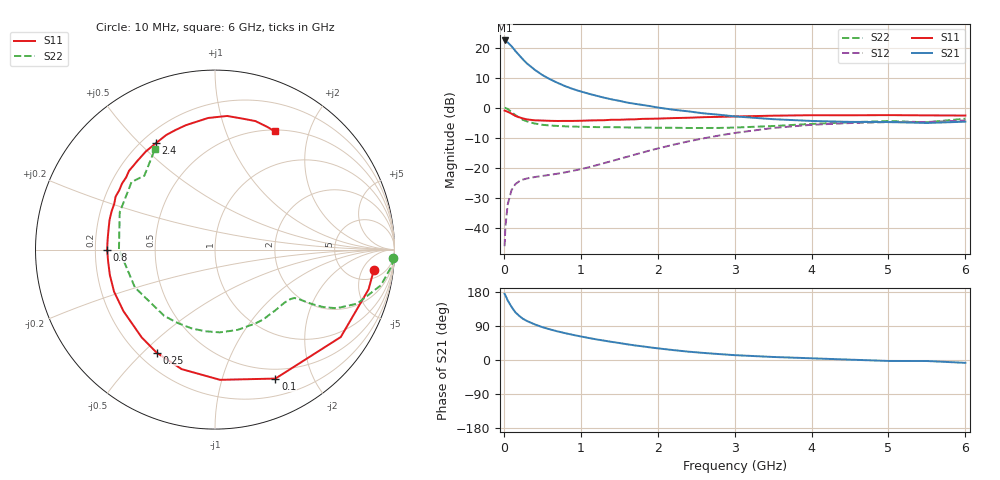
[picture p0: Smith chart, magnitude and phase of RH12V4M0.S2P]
! SIEMENS Small Signal Semiconductors
! BFR106
! Si NPN RF Bipolar Junction Transistor in SOT23
! VCE = 12 V  IC = 4 mA
! Common Emitter S-Parameters:  August  1996
# GHz  S  MA  R  50
!  f  S11  S21  S12  S22
! GHz  MAG  ANG  MAG  ANG  MAG  ANG  MAG  ANG
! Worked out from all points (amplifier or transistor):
!   36 points, 10 MHz to 6 GHz, reference 50 ohm
!   highest |S21| = 22.4 dB at 10 MHz (marker M1)
!   |S21| within 3 dB of that: start of sweep to 134.2 MHz
!   unconditionally stable (mu >= 1): 673 MHz to 1.807 GHz; 4.845 GHz to end of sweep
!   at 250 MHz: K = 0.44, MSG = 20.0 dB, |S12| = -24.0 dB
!   at 1.4 GHz: K = 1.14, MAG = 8.1 dB, |S12| = -17.8 dB
!   at 6 GHz: K = 1.02, MAG = -1.0 dB, |S12| = -4.3 dB
!   S11 on the Smith chart (normalised r, x): 10 MHz: 8, -9; 100 MHz: 0.39, -1.50; 250 MHz: 0.27, -0.55; 800 MHz: 0.25, -0.00; 2.4 GHz: 0.26, +0.56; 6 GHz: 0.52, +1.50
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0.01  0.8926 -7.2  13.19 174.6  0.0049 87.8  0.9945 -2.6
0.02  0.8838 -14.5  12.98 170.8  0.0101 82.2  0.9895 -5.2
0.05  0.8534 -34.8  12.21 157.3  0.0242 71.4  0.9459 -12.1
0.1  0.7935 -64.9  10.6 140.1  0.0422 58.6  0.8475 -20.8
0.15  0.7261 -87.8  8.806 125.8  0.0531 48.7  0.7512 -25.8
0.2  0.6914 -105.6  7.473 116.5  0.0592 43.7  0.6807 -28.0
0.25  0.6596 -119.6  6.338 108.5  0.0633 39.9  0.6249 -29.2
0.3  0.6372 -129.9  5.463 103.0  0.0659 38.4  0.5906 -29.8
0.4  0.6146 -146.1  4.293 94.1  0.0696 37.6  0.5438 -30.5
0.5  0.6093 -157.4  3.5 86.7  0.0726 38.9  0.5174 -31.4
0.6  0.6027 -166.4  2.976 80.8  0.0758 41.5  0.5038 -33.1
0.8  0.601 -180.0  2.274 70.7  0.0835 47.6  0.4877 -37.2
1.1  0.6104 164.2  1.712 58.3  0.101 57.5  0.4767 -45.4
1.3  0.6166 155.6  1.469 51.2  0.1186 62.4  0.4724 -51.7
1.6  0.6354 144.6  1.217 41.6  0.1513 66.9  0.4683 -62.2
2.2  0.6691 125.1  0.924 26.2  0.2402 66.3  0.4618 -86.8
2.4  0.6782 119.0  0.866 22.0  0.2742 64.0  0.4581 -96.9
3.5  0.7343 93.0  0.642 8.0  0.458 43.9  0.4936 -154.7
4.5  0.7457 77.9  0.579 0.9  0.5533 22.5  0.5701 158.6
5  0.7507 72.5  0.575 -2.5  0.5738 13.7  0.5984 141.0
5.5  0.7429 66.8  0.555 -2.7  0.5771 9.1  0.5697 133.7
6  0.7382 63.3  0.583 -7.5  0.6116 0.7  0.6544 120.6
